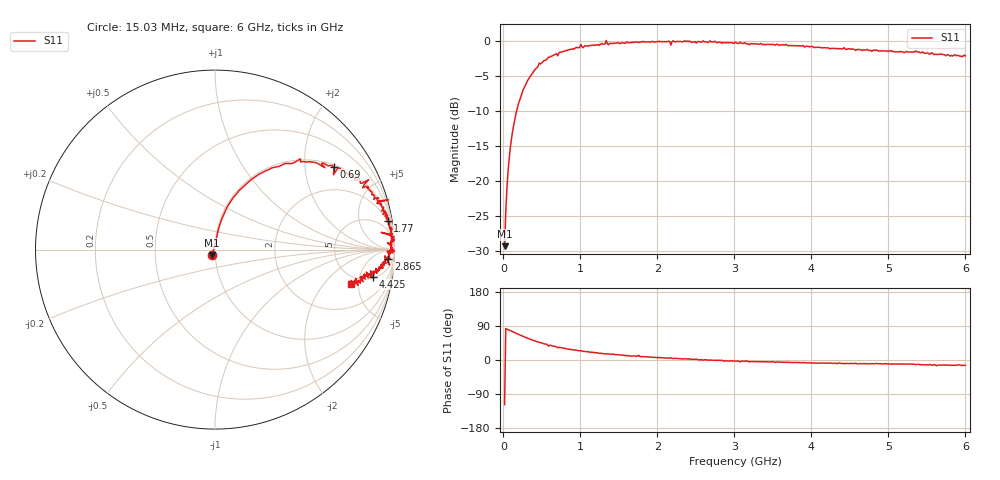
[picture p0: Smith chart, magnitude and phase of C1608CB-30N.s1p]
!	Network	Analyzer	HP8753E.07.74:	Oct	30	2002	Serial	No.	JP38451487
!	Hewlett-Packard
!	28	Aug	2009	8:02:50
!	Frequency	S11
#	HZ	S	RI	R	50
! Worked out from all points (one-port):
!   400 points, 15.03 MHz to 6 GHz, reference 50 ohm
!   lowest |S11| = -29.3 dB at 15.03 MHz (marker M1), VSWR 1.07, Z = 48.3 - j2.93 ohm
!   |S11| at or under -10 dB: start of sweep to 171.9 MHz
!   S11 on the Smith chart (normalised r, x): 15.03 MHz: 0.97, -0.06; 690 MHz: 1.07, +2.84; 1.77 GHz: 2, +12; 2.865 GHz: 16, -26; 4.425 GHz: 5.49, -8.18; 6 GHz: 4.08, -3.96
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1.502992e7  -0.0159 -0.0303
4.502978e7  0.0129 0.087
7.502962e7  0.0284 0.142
1.200294e8  0.0597 0.22
1.95029e8  0.134 0.329
4.650277e8  0.476 0.506
6.900266e8  0.664 0.46
7.650262e8  0.703 0.443
1.005025e9  0.857 0.39
1.320023e9  0.91 0.271
1.335023e9  0.966 0.277
1.365023e9  0.901 0.258
1.515022e9  0.928 0.216
1.740021e9  0.963 0.168
1.755021e9  0.948 0.214
1.770021e9  0.963 0.16
2.145019e9  0.991 0.0845
2.175019e9  0.926 0.0958
2.205019e9  0.997 0.0668
2.265019e9  0.99 0.0692
2.835016e9  0.959 -0.00806
2.865016e9  0.965 -0.0541
3.015015e9  0.977 -0.0495
3.765011e9  0.916 -0.1
4.425008e9  0.881 -0.15
4.515007e9  0.865 -0.136
5.265004e9  0.817 -0.155
6e9  0.755 -0.191
